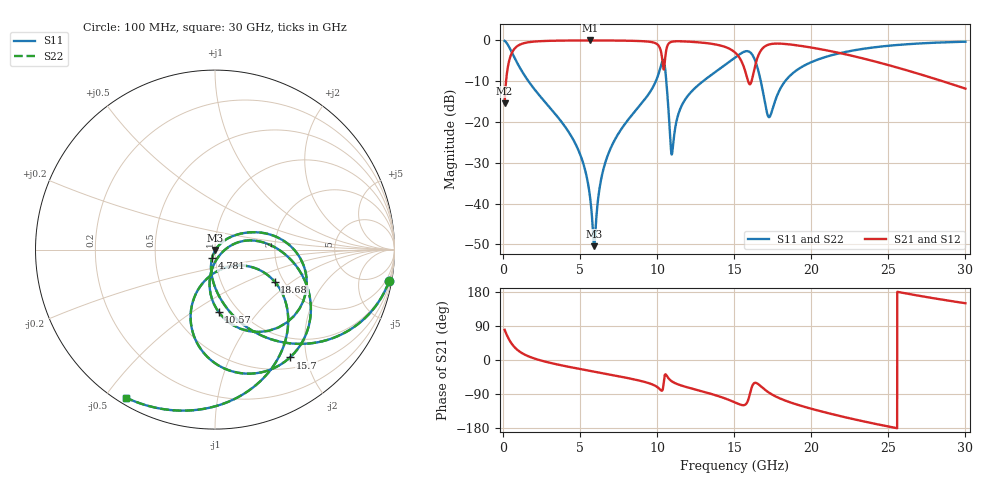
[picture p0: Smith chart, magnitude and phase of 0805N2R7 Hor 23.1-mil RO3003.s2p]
# GHz S MA R 50
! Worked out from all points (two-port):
!   3201 points, 100 MHz to 30 GHz, reference 50 ohm
!   highest |S21| = -0.03 dB at 5.669 GHz (marker M1); lowest = -15.4 dB at 100 MHz (marker M2)
!   |S21| within 3 dB of the highest: 576.6 MHz to 10.26 GHz (9.687 GHz wide, 179 % of centre); 16.65 GHz to 21.74 GHz (5.097 GHz wide, 26.6 % of centre)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
!   lowest |S11| = -50.4 dB at 5.912 GHz (marker M3), VSWR 1.01, Z = 50.3 - j0.16 ohm
!   |S11| at or under -10 dB: 1.644 GHz to 9.914 GHz (8.269 GHz wide, 143 % of centre); 10.59 GHz to 12.98 GHz (2.386 GHz wide, 20.2 % of centre); 16.72 GHz to 18.31 GHz (1.581 GHz wide, 9.03 % of centre)
!   |S22| runs from -50.4 to -0.1 dB; largest |S21 - S12| = 0
!   S11 on the Smith chart (normalised r, x): 100 MHz: 1, -11; 4.781 GHz: 0.96, -0.09; 10.57 GHz: 0.81, -0.64; 15.7 GHz: 0.66, -1.72; 18.68 GHz: 1.80, -0.75; 30 GHz: 0.03, -0.57
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0.1  0.9855 -10.3  0.1693 79.7  0.1693 79.7  0.9855 -10.3
0.5298125  0.7374 -45.2  0.6748 44.7  0.6748 44.7  0.7374 -45.2
1.389438  0.3726 -75.3  0.9267 14.6  0.9267 14.6  0.3726 -75.3
4.781219  0.05006 -109.2  0.996 -22.1  0.996 -22.1  0.05006 -109.2
5.089563  0.03609 -110.2  0.9965 -24.5  0.9965 -24.5  0.03609 -110.2
5.668875  0.01097 -103.6  0.9968 -28.9  0.9968 -28.9  0.01097 -103.6
5.911812  0.003005 -32.1  0.9968 -30.7  0.9968 -30.7  0.003005 -32.1
6.892906  0.04353 47.2  0.9953 -38.2  0.9953 -38.2  0.04353 47.2
10.06978  0.3785 8.2  0.8711 -73.3  0.8711 -73.3  0.3785 8.2
10.31272  0.5425 -19.5  0.6196 -81.0  0.6196 -81.0  0.5425 -19.5
10.57434  0.3474 -86.8  0.7333 -38.8  0.7333 -38.8  0.3474 -86.8
10.98547  0.04329 -19.6  0.965 -57.2  0.965 -57.2  0.04329 -19.6
11.90116  0.1988 14.9  0.9672 -71.5  0.9672 -71.5  0.1988 14.9
15.05  0.614 -29.7  0.7102 -112.0  0.7102 -112.0  0.614 -29.7
15.70406  0.7318 -55.2  0.4244 -118.1  0.4244 -118.1  0.7318 -55.2
16.04978  0.7094 -76.7  0.2919 -84.3  0.2919 -84.3  0.7094 -76.7
16.47959  0.4826 -104.7  0.5911 -61.6  0.5911 -61.6  0.4826 -104.7
17.24578  0.1146 -70.7  0.8883 -85.9  0.8883 -85.9  0.1146 -70.7
18.67537  0.3772 -28.2  0.8878 -112.4  0.8878 -112.4  0.3772 -28.2
20.03956  0.5443 -41.7  0.8138 -129.1  0.8138 -129.1  0.5443 -41.7
25.01978  0.8586 -86.6  0.4966 -175.6  0.4966 -175.6  0.8586 -86.6
30  0.9622 -120.9  0.2563 149.9  0.2563 149.9  0.9622 -120.9
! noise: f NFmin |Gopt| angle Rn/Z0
0.1  0.0009338  0.9356  1.297  0.003229
3.417  0.00638  0.7064  18.35  0.004164
6.743  0.01151  0.6874  34.78  0.006535
10.06  0.05755  0.8975  51.13  0.09988
13.39  0.03581  0.7976  66.34  0.02579
16.7  0.1657  0.9422  81.84  0.3665
20.03  0.05577  0.8124  95.24  0.02855
23.35  0.05688  0.7943  107.7  0.02038
26.67  0.06927  0.8132  120  0.01997
30  0.09175  0.8474  132.5  0.02152
